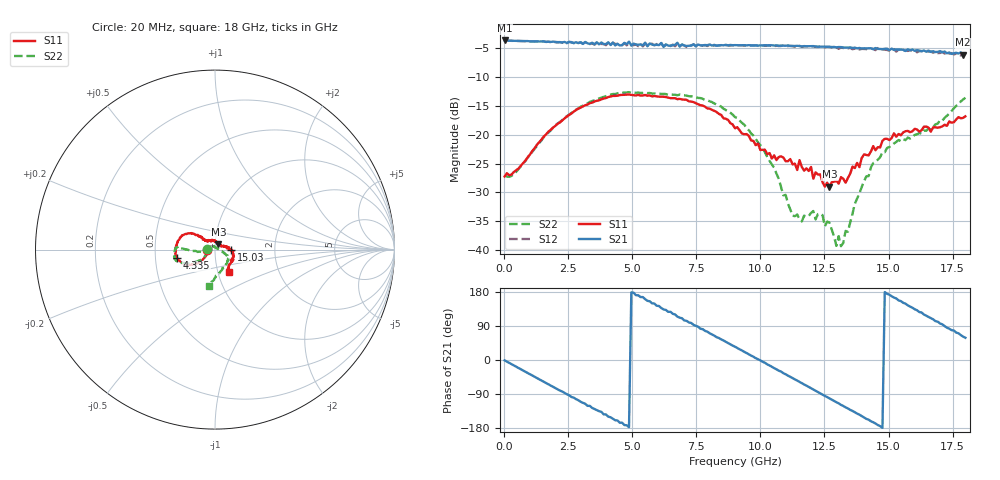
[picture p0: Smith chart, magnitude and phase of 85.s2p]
!Agilent Technologies,N5230A,US43500223,A.07.50.48
!Agilent N5230A: A.07.50.48
!Date: Wednesday, January 13, 2016 17:43:18
!Correction: S11(Full 2 Port(1,2))
!S21(Full 2 Port(1,2))
!S12(Full 2 Port(1,2))
!S22(Full 2 Port(1,2))
!S2P File: Measurements: S11, S21, S12, S22:
# Hz S  dB  R 50
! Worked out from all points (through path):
!   201 points, 20 MHz to 18 GHz, reference 50 ohm
!   highest |S21| = -3.72 dB at 20 MHz (marker M1); lowest = -6.2 dB at 17.91 GHz (marker M2)
!   group delay of S21, straight-line fit = 101 ps
!   lowest |S11| = -29.0 dB at 12.7 GHz (marker M3), VSWR 1.07, Z = 51.8 + j3.12 ohm
!   |S11| at or under -10 dB: start of sweep to end of sweep
!   |S22| runs from -39.3 to -12.7 dB; largest |S21 - S12| = 0.055
!   S11 on the Smith chart (normalised r, x): 20 MHz: 0.92, -0.00; 4.335 GHz: 0.65, -0.07; 15.03 GHz: 1.20, -0.00; 18 GHz: 1.13, -0.28
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2e7  -27.23 -178.6  -3.72 -0.9  -3.74 -0.9  -27.10 178.9
1.5483e9  -20.34 -140.2  -3.88 -57.6  -3.88 -58.1  -20.43 -144.1
2.3574e9  -17.20 -143.8  -3.98 -86.8  -4.03 -87.1  -17.10 -149.0
3.0766e9  -15.13 -150.9  -4.33 -113.0  -4.26 -113.8  -14.99 -154.2
4.3352e9  -13.31 -167.2  -4.58 -158.9  -4.33 -159.5  -12.99 -163.9
4.8746e9  -13.06 -174.0  -3.92 -177.2  -4.13 -177.0  -12.66 -168.4
6.0433e9  -13.44 169.3  -4.53 142.5  -4.79 140.4  -12.94 -177.2
6.7625e9  -13.87 160.3  -4.12 114.4  -4.32 113.5  -13.19 178.1
7.5716e9  -14.74 151.6  -4.43 87.8  -4.39 86.2  -13.66 177.0
9.01e9  -18.92 141.3  -4.53 35.1  -4.53 32.9  -16.97 -178.1
1.01787e10  -22.63 138.8  -4.55 -7.3  -4.64 -10.2  -23.07 -169.0
1.12575e10  -25.15 110.6  -4.66 -47.9  -4.72 -50.8  -34.02 166.3
1.19767e10  -25.59 91.3  -4.72 -74.5  -4.79 -76.6  -33.55 122.7
1.20666e10  -27.63 82.7  -4.70 -77.8  -4.74 -80.3  -33.21 115.3
1.26959e10  -29.02 58.1  -4.81 -101.3  -4.86 -104.6  -35.23 96.2
1.31454e10  -27.36 44.1  -4.87 -118.4  -4.94 -120.5  -39.29 52.7
1.33252e10  -28.32 26.5  -4.95 -124.9  -5.14 -127.7  -36.65 25.1
1.41343e10  -23.51 5.9  -5.09 -155.3  -5.22 -157.7  -27.23 -17.0
1.50333e10  -20.94 -0.3  -5.40 172.2  -5.49 167.8  -22.14 -27.5
1.65616e10  -18.79 -36.4  -5.48 113.9  -5.66 110.4  -18.93 -62.9
1.79101e10  -17.11 -58.9  -6.21 61.8  -6.04 58.7  -13.94 -99.8
1.8e10  -16.84 -58.1  -5.98 58.7  -6.28 54.9  -13.63 -100.0
